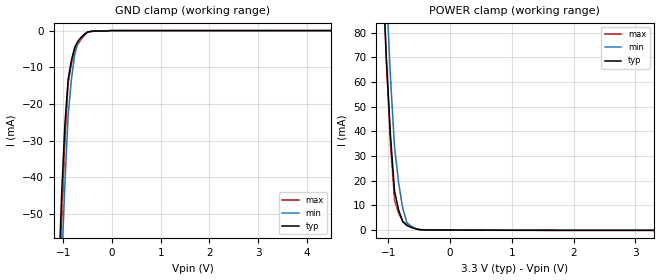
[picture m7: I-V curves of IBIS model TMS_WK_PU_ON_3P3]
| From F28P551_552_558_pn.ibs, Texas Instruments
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|TMS_WK_PD_ON_3P3; WEAK_PULLDOWN_ON
|   Model Cell TMS_WK_PU_ON_3P3
|TMS_WK_PU_ON_3P3
[Model]   TMS_WK_PU_ON_3P3
Model_type   Input
Polarity   Non-Inverting
Vinl =  0.8
Vinh =  2
C_comp   1.26765p   1.03155p   1.45072p
[Model Spec]
Vinl   0.8   0.8   0.8
Vinh   2   2   2
[Temperature Range]   25   155   -40
[Voltage Range]   3.3   2.97   3.63
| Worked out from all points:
|   GND clamp passes 1 mA (typ) near -0.57 V on its own axis
|   POWER clamp passes 1 mA (typ) near -0.62 V on its own axis
| Nom Voltages:
|   BIASFET=3.3, VDD=1.2, VDDS=3.3, VSS=0
| Min Voltages:
|   BIASFET=2.97, VDD=1.08, VDDS=2.97, VSS=0
| Max Voltages:
|   BIASFET=3.63, VDD=1.32, VDDS=3.63, VSS=0
[POWER_clamp]
|   voltage   I(typ)   I(min)   I(max)
-3.3V     1.919A     2.431A     2.069A
-1.1V     109.6mA    140.7mA    112.7mA
-1.033V   69.94mA    97.94mA    68.79mA
-966.7mV  38.68mA    62.24mA    35.25mA
-900mV    15.78mA    33.62mA    12.06mA
-833.3mV  8.07mA     18.99mA    6.791mA
-766.7mV  3.419mA    8.778mA    3.538mA
-700mV    1.823mA    2.989mA    2.306mA
-566.7mV  559.2uA    664.6uA    706.6uA
-500mV    180.3uA    246.8uA    210.6uA
-366.7mV  40uA       41.62uA    52.55uA
3.3V      -108.8uA   -62.86uA   -174uA
[GND_clamp]
|   voltage   I(typ)   I(min)   I(max)
-3.3V     -1.48A     -1.41A     -2.182A
-1.1V     -69.77mA   -89.94mA   -82.81mA
-1.033V   -44.51mA   -64.23mA   -52.89mA
-966.7mV  -25.68mA   -41.95mA   -30.11mA
-900mV    -13.28mA   -23.08mA   -14.48mA
-833.3mV  -8.104mA   -13.36mA   -9.06mA
-766.7mV  -4.652mA   -6.722mA   -5.47mA
-700mV    -2.919mA   -3.153mA   -3.707mA
-566.7mV  -1.003mA   -1.018mA   -1.284mA
-500mV    -378.3uA   -440.9uA   -479.8uA
-33.33mV  0A         0A         0A
6.6V      0A         0A         0A
